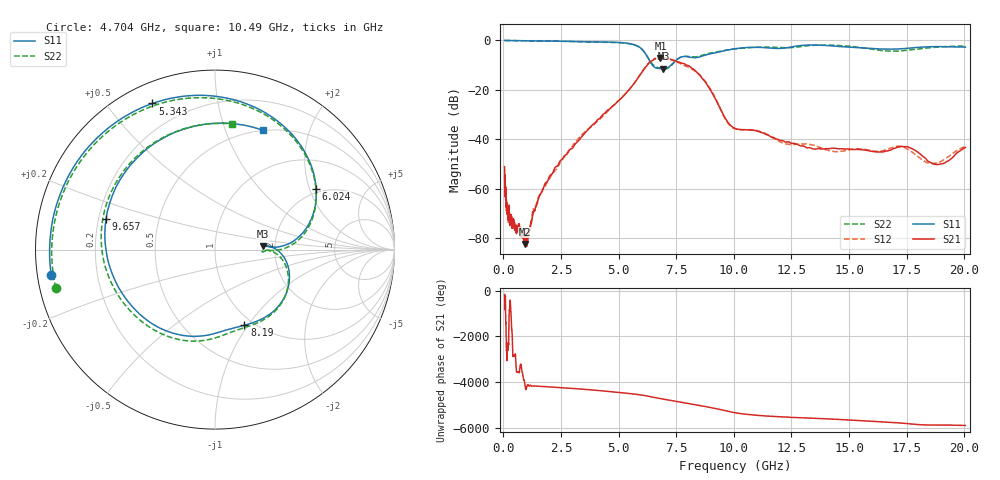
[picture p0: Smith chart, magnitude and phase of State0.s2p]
# Hz S DB R 50
!freq MagS11 AngS11 MagS21 AngS21 MagS12 AngS12 MagS22 AngS22
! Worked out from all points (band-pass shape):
!   1601 points, 50 MHz to 20.05 GHz, reference 50 ohm
!   highest |S21| = -7.20 dB at 6.816 GHz (marker M1); lowest = -82.4 dB at 929 MHz (marker M2)
!   |S21| within 3 dB of the highest: 6.226 GHz to 8.027 GHz (1.801 GHz wide, 25.3 % of centre)
!   lowest |S11| = -11.4 dB at 6.945 GHz (marker M3), VSWR 1.73, Z = 86.5 + j3.45 ohm
!   |S11| at or under -10 dB: 6.466 GHz to 7.273 GHz (806.8 MHz wide, 11.7 % of centre)
!   |S22| runs from -11.6 to 0.0 dB; largest |S21 - S12| = 0.028
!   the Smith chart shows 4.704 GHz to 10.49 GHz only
!   S11 on the Smith chart (normalised r, x): 4.704 GHz: 0.04, -0.08; 5.343 GHz: 0.09, +0.66; 6.024 GHz: 1.85, +2.22; 8.19 GHz: 0.91, -0.96; 9.657 GHz: 0.23, +0.13; 10.49 GHz: 0.50, +1.36
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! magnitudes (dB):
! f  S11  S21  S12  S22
! 50 MHz  0.0  -51.1  -57.1  0.0
! 66.22 MHz  0.0  -60.2  -57.6  0.0
! 116.6 MHz  0.0  -63.5  -61.1  0.0
! 135.9 MHz  0.0  -67.2  -68.8  0.0
! 241.2 MHz  0.0  -66.9  -70.0  0.0
! 369.6 MHz  0.0  -75.6  -73.9  0.0
! 929 MHz  -0.1  -82.4  -79.9  -0.1
! 1.005 GHz  -0.1  -80.5  -82.0  -0.1
! 2.722 GHz  -0.3  -46.2  -46.1  -0.4
! 4.704 GHz  -0.7  -26.8  -27.0  -0.8
! 5.343 GHz  -1.1  -21.1  -21.1  -1.2
! 6.024 GHz  -3.6  -12.7  -12.5  -3.7
! 6.816 GHz  -11.4  -7.2  -7.0  -11.3
! 6.945 GHz  -11.4  -7.3  -7.0  -11.6
! 7.402 GHz  -8.8  -8.0  -8.2  -8.9
! 8.19 GHz  -6.9  -11.3  -11.6  -6.7
! 9.657 GHz  -4.0  -31.9  -32.3  -3.9
! 10.49 GHz  -2.9  -36.1  -36.1  -3.0
! 13.48 GHz  -1.8  -44.0  -42.4  -2.0
! 17.45 GHz  -3.2  -43.0  -43.6  -4.0
! 18.6 GHz  -2.5  -49.7  -49.8  -2.8
! 20.05 GHz  -2.7  -43.4  -43.1  -2.2
